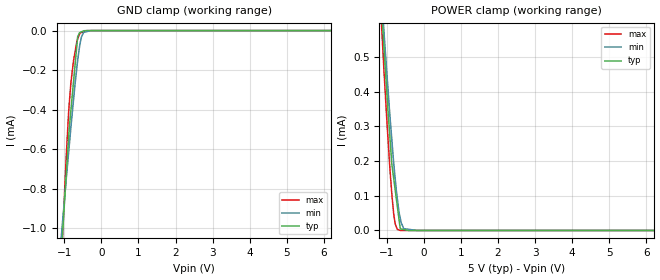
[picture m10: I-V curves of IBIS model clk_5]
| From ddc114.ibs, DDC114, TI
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|   clk_5 Model
[Model]   clk_5
Model_type   Input
Vinl = 1
Vinh = 4
|   typ   min   max
|   (nom PVT)   (fast PVT)   (slow PVT)
|C_comp from frequency sweep method (F=19.2MHz)
|Average
C_comp   4.789e-13   4.180e-13   5.393e-13
|C_comp from LC tank measurement(L=1nH)
|Average
|Resonant Frequency(Hz)   5.150e+10   6.030e+10   3.004e+10
|C_comp   9.560e-15   6.973e-15   2.810e-14
| Where nom  PVT is Nominal Process, 5V, 27C
|   Fast PVT is Strong Process,  5.25V, -40C
|   Slow PVT is Weak Process,   4.75V, 87C
[Model Spec]
|Subparameter   typ   min   max
Vinl   1.0   0.95   1.05
Vinh   4.0   3.8   4.2
[Voltage Range]   5   4.75   5.25
|Ambient Temperature   25   85   -40
|Junction Temperature
[Temperature Range]   27   87   -40
[Power Clamp Reference]   5   4.75   5.25
[GND Clamp Reference]   0   0   0
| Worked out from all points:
|   GND clamp passes 1 mA (typ) near -1.04 V on its own axis
|   POWER clamp passes 1 mA (typ) near -1.34 V on its own axis
[GND Clamp]
|   Voltage   I(typ)   I(min)   I(max)
-5V       -13.83mA   -10.04mA   -20.04mA
-1.08V    -1.124mA   -1.037mA   -1.186mA
-1.034V   -986.1uA   -938uA     -985.1uA
-950.3mV  -734.7uA   -756.5uA   -643.9uA
-887.2mV  -553.6uA   -624.3uA   -425.3uA
-824.3mV  -406.6uA   -493.1uA   -267.8uA
-750.8mV  -257uA     -348.7uA   -151.3uA
-640mV    -31.43uA   -150.3uA   -41.3uA
-584.3mV  -10.56uA   -74.07uA   -16.34uA
-536.7mV  -6.343uA   -31.85uA   -9.65uA
-475mV    -859.4nA   -8.646uA   -5.651uA
10V       0A         0A         0A
[POWER Clamp]
|   Voltage   I(typ)   I(min)   I(max)
-5V       8.406mA    7.827mA    9.173mA
-1.306V   939.1uA    952.3uA    920.1uA
-1.088V   544.8uA    590.4uA    482.5uA
-1.08V    531.2uA    578.3uA    467uA
-992.2mV  385.4uA    443uA      304.8uA
-865mV    191.4uA    261.5uA    105.1uA
-813.7mV  149.3uA    193.8uA    47.68uA
-719.2mV  71.78uA    93.94uA    3.526uA
-640.5mV  7.165uA    36.86uA    168.1nA
-541.5mV  2.737uA    5.32uA     142.2nA
-190mV    0A         0A         49.89nA
10V       0A         0A         0A
